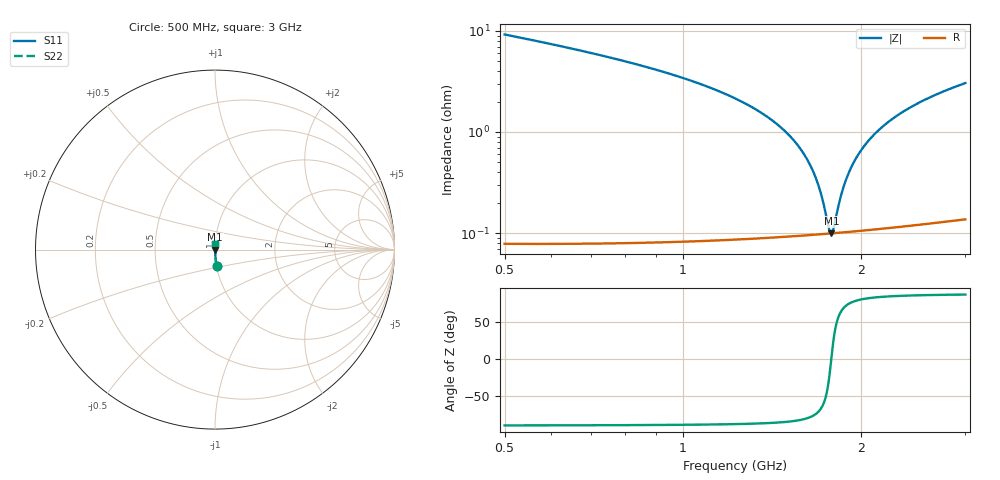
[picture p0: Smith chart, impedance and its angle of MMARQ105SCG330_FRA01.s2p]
! MMARQ105SCG330_FRA01  S-PARAMETER MODEL  ( General Type )
! Model Generated by TAIYO YUDEN Corporation (http://www.ty-top.com)
! Version 1.0
! TAIYO YUDEN Control No. 200326
! Copyright(c) 2020 TAIYO YUDEN CO.,LTD. All Rights Reserved.
! Product Description (link to TY-COMPAS)
! https://ds.yuden.co.jp/TYCOMPAS/or/detail?pn=MMARQ105SCG330JFRA01&u=M
! Products Name : Multilayer Ceramic Capacitors
! Characteristics :
!  Capacitance : 33 pF , Rated Voltage : 250V , TCC : CG / C0G
!  Case Size : 1.0 x 0.5 / 0.039 x 0.02 [mm/inch] , Thickness : 0.5 / 0.02 [mm/inch]
!  (Conditions: Temperature = 25 degC , DC Bias Current/Voltage = 0A / 0V)
! External Node Assignments :
!  1  o---| |---o  2
! GND o---------o GND
! Frequency Range : 500MHz  -  3GHz  [ 401 STEP ]
# MHz S RI R 50
! Freq[MHz].  S11 Real  S11 Imag  S21 Real  S21 Imag  S12 Real  S12 Imag  S22 Real  S22 Imag
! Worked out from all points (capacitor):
!   401 points, 500 MHz to 3 GHz, reference 50 ohm
!   read as one part in series: C = 31.8 pF near 512.5 MHz
!   lowest |Z| = 99.2 mohm at 1.781 GHz (marker M1)
!   series resonance near 1.781 GHz, so ESL is about 250 pH
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500  0.00919 -0.0913  0.9908 0.0913  0.9908 0.0913  0.00919 -0.0913
918.75  0.0024 -0.0398  0.9976 0.0398  0.9976 0.0398  0.0024 -0.0398
1162.5  0.00146 -0.0246  0.9985 0.0246  0.9985 0.0246  0.00146 -0.0246
1337.5  0.00115 -0.0163  0.9989 0.0163  0.9989 0.0163  0.00115 -0.0163
1493.75  0.00102 -0.00989  0.999 0.00989  0.999 0.00989  0.00102 -0.00989
1606.25  0.00098 -0.00579  0.999 0.00579  0.999 0.00579  0.00098 -0.00579
1650  0.000975 -0.00428  0.999 0.00428  0.999 0.00428  0.000975 -0.00428
1687.5  0.000976 -0.00302  0.999 0.00302  0.999 0.00302  0.000976 -0.00302
1718.75  0.000979 -0.00199  0.999 0.00199  0.999 0.00199  0.000979 -0.00199
1750  0.000984 -0.000979  0.999 0.000979  0.999 0.000979  0.000984 -0.000979
1768.75  0.000988 -0.000383  0.999 0.000383  0.999 0.000383  0.000988 -0.000383
1781.25  0.000991 1.15e-05  0.999 -1.15e-05  0.999 -1.15e-05  0.000991 1.15e-05
1800  0.000997 0.000597  0.999 -0.000597  0.999 -0.000597  0.000997 0.000597
1837.5  0.00101 0.00175  0.999 -0.00175  0.999 -0.00175  0.00101 0.00175
1868.75  0.00102 0.00269  0.999 -0.00269  0.999 -0.00269  0.00102 0.00269
1931.25  0.00105 0.00454  0.9989 -0.00454  0.9989 -0.00454  0.00105 0.00454
1975  0.00108 0.00579  0.9989 -0.00579  0.9989 -0.00579  0.00108 0.00579
2031.25  0.00112 0.00737  0.9989 -0.00737  0.9989 -0.00737  0.00112 0.00737
2168.75  0.00122 0.0111  0.9988 -0.0111  0.9988 -0.0111  0.00122 0.0111
2350  0.0014 0.0157  0.9986 -0.0157  0.9986 -0.0157  0.0014 0.0157
2587.5  0.00169 0.0213  0.9983 -0.0213  0.9983 -0.0213  0.00169 0.0213
3000  0.00229 0.0303  0.9977 -0.0303  0.9977 -0.0303  0.00229 0.0303
